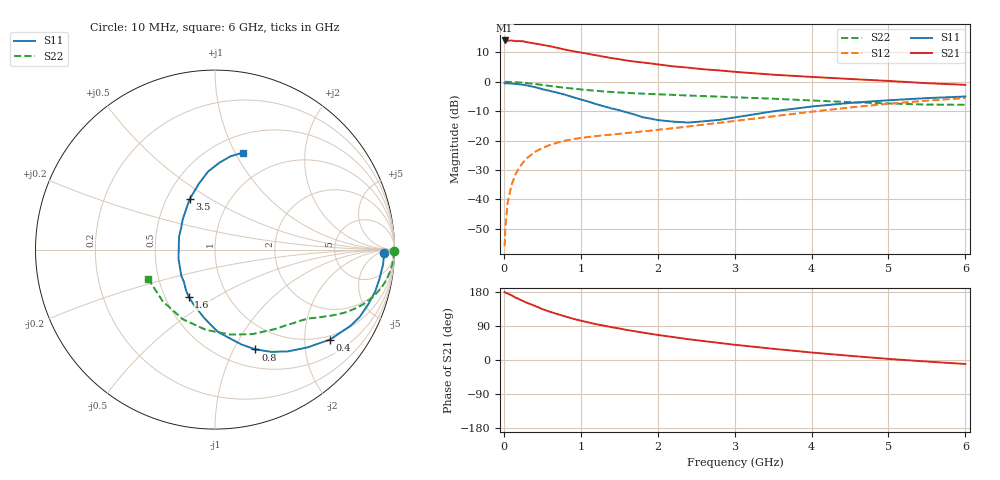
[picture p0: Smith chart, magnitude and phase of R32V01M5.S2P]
! SIEMENS Small Signal Semiconductors
! BFR181
! Si NPN RF Bipolar Junction Transistor in SOT23
! VCE = 2 V  IC = 1.5 mA
! Common Emitter S-Parameters:  May  1996
# GHz  S  MA  R  50
!  f  S11  S21  S12  S22
! GHz  MAG  ANG  MAG  ANG  MAG  ANG  MAG  ANG
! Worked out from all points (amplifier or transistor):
!   36 points, 10 MHz to 6 GHz, reference 50 ohm
!   highest |S21| = 14.1 dB at 10 MHz (marker M1)
!   |S21| within 3 dB of that: start of sweep to 777 MHz
!   unconditionally stable (mu >= 1): 1.728 GHz to 3.515 GHz
!   at 250 MHz: K = 0.20, MSG = 20.6 dB, |S12| = -27.5 dB
!   at 1.4 GHz: K = 0.89, MSG = 13.0 dB, |S12| = -18.0 dB
!   at 6 GHz: K = 0.87, MSG = 2.2 dB, |S12| = -5.5 dB
!   S11 on the Smith chart (normalised r, x): 10 MHz: 30, -9; 400 MHz: 0.89, -2.64; 800 MHz: 0.70, -1.22; 1.6 GHz: 0.66, -0.38; 3.5 GHz: 0.65, +0.41; 6 GHz: 0.68, +1.07
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0.01  0.9404 -1.1  5.041 179.3  0.0016 90.2  0.9976 -0.5
0.02  0.9422 -2.0  4.975 177.9  0.0034 81.6  0.9946 -1.0
0.05  0.94 -5.2  4.992 175.3  0.0089 86.2  0.996 -2.4
0.1  0.9309 -10.1  5.038 170.6  0.0176 83.9  0.9915 -4.7
0.15  0.9224 -14.7  4.912 164.9  0.0264 80.4  0.9832 -7.0
0.25  0.8894 -24.9  4.887 155.5  0.0424 74.5  0.9621 -11.3
0.4  0.8136 -38.0  4.48 143.2  0.0637 67.6  0.9183 -16.8
0.5  0.75 -46.6  4.247 134.3  0.0747 63.2  0.8836 -20.0
0.6  0.6975 -54.4  4.019 127.3  0.0843 59.7  0.8483 -22.7
0.8  0.5998 -68.0  3.512 114.8  0.0998 54.2  0.7893 -26.8
0.9  0.5466 -74.7  3.31 108.9  0.1057 52.4  0.7649 -28.3
1.1  0.4594 -87.9  2.983 99.1  0.115 50.3  0.7195 -31.1
1.2  0.416 -93.7  2.821 94.5  0.1192 49.5  0.7015 -32.4
1.4  0.3522 -105.2  2.525 86.6  0.1262 48.9  0.671 -34.6
1.6  0.3009 -119.1  2.294 79.2  0.1345 49.0  0.6478 -36.4
1.9  0.2375 -142.3  2.057 69.3  0.1474 50.1  0.6201 -39.7
2.2  0.2098 -165.4  1.83 60.6  0.162 51.2  0.5988 -43.3
2.8  0.2248 146.8  1.56 45.1  0.2007 53.2  0.5589 -51.9
3.5  0.3143 116.8  1.32 29.6  0.2584 52.1  0.5152 -66.1
4.5  0.4371 95.0  1.116 11.0  0.3651 45.1  0.4501 -96.4
5.5  0.5274 80.5  0.946 -4.1  0.4773 32.5  0.4092 -135.4
6  0.5614 74.1  0.886 -10.5  0.5282 25.0  0.4061 -156.0
